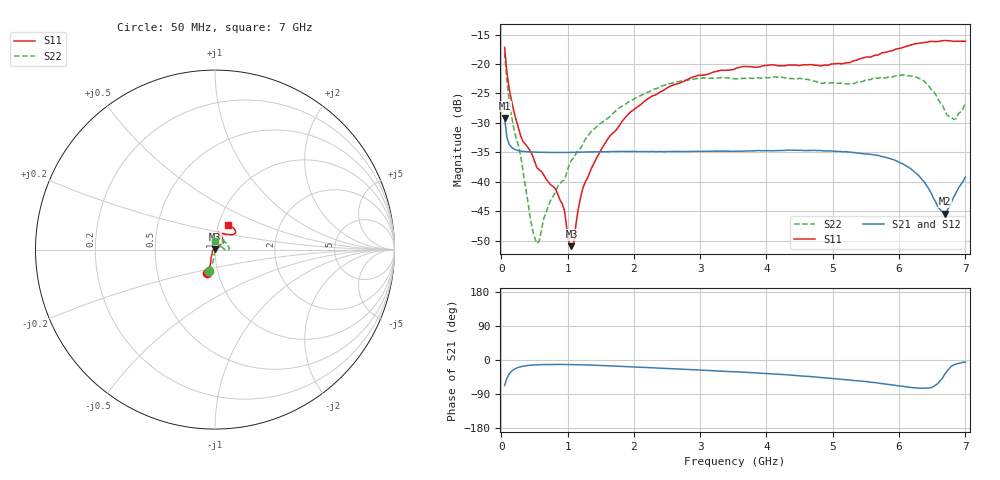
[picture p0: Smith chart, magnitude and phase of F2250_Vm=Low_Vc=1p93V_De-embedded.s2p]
! Integrated Device Technology
! Corporate Headquarters
! 6024 Silver Creek Valley Road
! San Jose, CA 95138  USA
! Phone:  1-408-284-8200
! Toll Free:  1-800-223-1366
! Webpage:  http://www.idt.com/
! Timing and RF Division
! 515 Groton Road, Suite 102
! Westford, MA 01886-6024
! Device:  F2250
! Description: Voltage Variable RF Attenuator
! Frequency:  50.0 -  6000.00 MHz
! Package:  3x3 mm Thin QFN Plastic Package: 16 pin
! Ports:  2 RF, 3 DC
!  Pin  1  = GND
!  Pin  2  = NC
!  Pin  3  = RF1  = Port 1
!  Pin  4  = NC
!  Pin  5  = GND
!  Pin  6  = GND
!  Pin  7  = GND
!  Pin  8  = GND
!  Pin  9  = NC
!  Pin 10  = RF2  = Port 2
!  Pin 11  = NC
!  Pin 12  = GND
!  Pin 13  = GND
!  Pin 14  = VCNTRL
!  Pin 15  = VDD
!  Pin 16  = VMODE
! Vcntrl:  1.930 Volts
! Vmode:  +0.000 Volts
! Vdd:  +3.30  Volts
! Current:  1.183 mA
! Data:  The device was measured on a the F2250 evaluation board which has
!  individual transmission lines to the RF pins.  Data was collected
!  using a calibrated network analyzer.  The evaluation board was
!  de-embedded using a TRL calibration technique.
!  The reference plane is the edge of the package pin.
! Misc:  SN 10
!  Action Tracker AT0258
! Date Measured:  2014-11-26
! Date:  2015-10-15  MJV
! Note:
!  Integrated Device Technology supplies this data as a sample of measured
!  data at the package pin for this product.  Your particular data for this
!  product may vary.
!  Data was taken at 25 degrees C.
!  Integrated Device Technology reserves the right to change this data at anytime.
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# GHz S dB R 50
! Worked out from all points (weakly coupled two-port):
!   201 points, 50 MHz to 7 GHz, reference 50 ohm
!   highest |S21| = -29.17 dB at 50 MHz (marker M1); lowest = -45.4 dB at 6.687 GHz (marker M2)
!   lowest |S11| = -51.0 dB at 1.058 GHz (marker M3), VSWR 1.01, Z = 49.9 + j0.242 ohm
!   |S11| at or under -10 dB: start of sweep to end of sweep
!   |S22| runs from -50.5 to -18.1 dB; largest |S21 - S12| = 5.5e-05
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0.05  -17.18 -108.6  -29.17 -67.2  -29.17 -67.2  -18.13 -106.6
0.1195  -24.19 -111.7  -33.64 -36.7  -33.64 -36.7  -26.32 -99.3
0.22375  -29.51 -122.0  -34.61 -21.9  -34.61 -21.8  -32.59 -97.4
0.29325  -32.22 -127.4  -34.79 -17.8  -34.79 -17.8  -35.68 -89.3
0.467  -35.43 -147.0  -34.95 -13.4  -34.95 -13.4  -47.97 -56.3
0.5365  -37.61 -155.2  -34.98 -12.7  -34.98 -12.7  -50.52 -29.0
0.71025  -40.05 -167.9  -35.02 -11.9  -35.02 -11.9  -44.11 20.6
0.91875  -43.74 158.3  -35.03 -11.8  -35.03 -11.8  -39.88 30.0
1.023  -50.47 143.6  -35.02 -12.0  -35.02 -12.0  -37.16 35.7
1.05775  -50.96 120.8  -35.02 -12.0  -35.02 -12.1  -36.36 36.5
1.0925  -50.52 87.9  -35.01 -12.1  -35.01 -12.2  -35.90 34.9
1.162  -44.57 55.6  -34.99 -12.4  -34.99 -12.4  -34.66 30.6
1.2315  -41.06 43.2  -34.97 -12.7  -34.97 -12.7  -33.59 28.0
1.6485  -32.09 41.7  -34.90 -15.5  -34.89 -15.4  -28.81 34.3
2.37825  -24.88 47.2  -34.87 -21.4  -34.87 -21.4  -23.99 40.3
3.525  -20.81 72.4  -34.83 -31.1  -34.83 -31.1  -22.51 65.4
4.7065  -20.17 72.3  -34.67 -44.4  -34.67 -44.4  -22.89 66.8
5.85325  -17.82 40.4  -36.04 -64.8  -36.04 -64.8  -22.20 13.6
6.33975  -16.41 40.9  -39.57 -74.5  -39.58 -74.6  -22.63 -0.5
6.68725  -15.99 48.8  -45.42 -38.0  -45.42 -37.8  -27.85 19.7
6.82625  -16.14 53.6  -42.56 -13.1  -42.52 -13.0  -29.43 52.2
7  -16.12 63.2  -39.20 -5.5  -39.16 -5.6  -26.46 90.4
